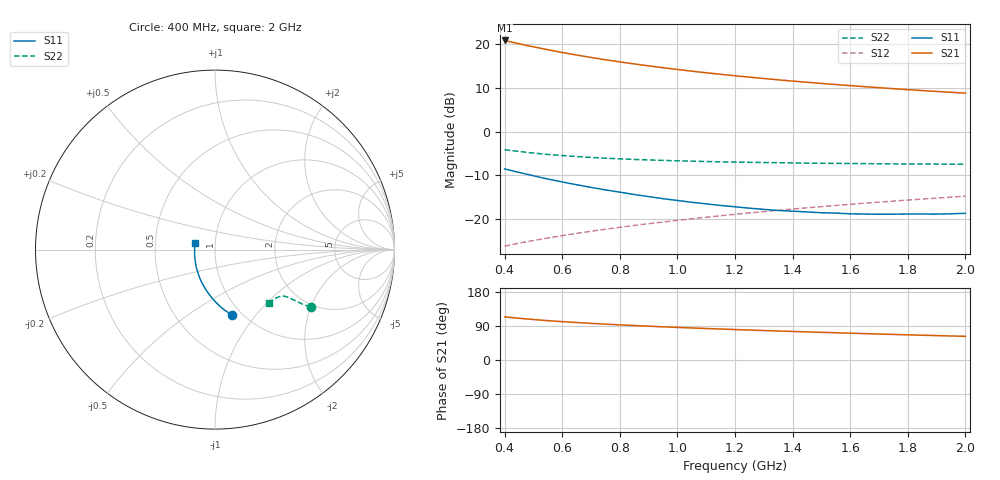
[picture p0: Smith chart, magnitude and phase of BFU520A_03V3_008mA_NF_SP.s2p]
! Filename:  P:\Prog\Test\Noise\ATS_data\Testdata_Net\06 Compressed Noise after Statistics\BFU520A_APG2013_30_A05_03p3V_008mA_NF_CM01_D.sf
! Date/Time: Wed 24/Apr/2013 20:06:16
! BFU520A_APG2013_30_A05_03p3V_1to20mA_NF_CM01_Bias5_R.sf
! Noise Parameter Data File
! BFU520A_APG2013_30_A05_03p3V_1to20mA_NF_CM01
! Date/time: Thu Apr 11 00:04:13 2013
! VAR V_out= 3.300000
! VAR I_out= 7.995000
! VAR V_in= 0.843200
! VAR I_in= 0.090005
! Device data file deembeded for feedlines and parallel
! Original file: \06 Compressed Noise after Statistics\BFU520A_APG2013_30_A05_03p3V_008mA_NF_CM01_R.sf
! Feed-files: PR017V01_150413_Feed1.s2p, PR017V01_150413_Feed2.s2p
! Parallel-file: PR017V01_150413_Par.s2p
# MHz S MA R 50
!  Freq-MHz  S11-mag  S11-arg  S21-mag  S21-arg  S12-mag  S12-arg  S22-mag  S22-arg
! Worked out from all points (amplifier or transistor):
!   37 points, 400 MHz to 2 GHz, reference 50 ohm
!   highest |S21| = 20.9 dB at 400 MHz (marker M1)
!   |S21| within 3 dB of that: start of sweep to 621.3 MHz
!   unconditionally stable (mu >= 1): 1.331 GHz to end of sweep
!   at 500 MHz: K = 0.78, MSG = 22.2 dB, |S12| = -24.9 dB
!   at 1.1 GHz: K = 0.98, MSG = 16.5 dB, |S12| = -19.6 dB
!   at 2 GHz: K = 1.01, MAG = 11.2 dB, |S12| = -14.8 dB
!   lowest NFmin = 0.77 dB at 420 MHz
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400  0.3744 -75.7  11.06 113.9  0.04886 66.5  0.621 -31.0
420  0.361 -77.8  10.67 112.3  0.05052 66.4  0.6089 -31.3
440  0.3475 -79.9  10.31 110.8  0.05208 66.4  0.598 -31.5
460  0.3356 -81.8  9.965 109.5  0.05367 66.4  0.5879 -31.7
480  0.324 -83.8  9.645 108.2  0.0552 66.5  0.5777 -31.9
500  0.3125 -85.8  9.341 106.9  0.05679 66.5  0.5693 -32.0
550  0.2868 -90.3  8.674 103.8  0.06059 66.8  0.5482 -32.2
600  0.2653 -94.5  8.057 101.2  0.06453 67.0  0.5323 -32.4
650  0.2468 -98.5  7.532 98.9  0.06843 67.3  0.5185 -32.6
700  0.2302 -102.5  7.069 96.7  0.07236 67.6  0.5068 -32.7
750  0.2154 -106.2  6.653 94.6  0.07633 67.9  0.4967 -32.9
800  0.2029 -110.2  6.288 92.7  0.08036 68.1  0.4884 -33.1
850  0.1907 -114.1  5.959 90.9  0.08437 68.3  0.4806 -33.3
950  0.1708 -121.6  5.39 87.5  0.09243 68.7  0.4684 -33.8
1050  0.1553 -128.9  4.923 84.5  0.1006 68.9  0.4587 -34.4
1150  0.1429 -136.9  4.533 81.7  0.1089 69.0  0.4511 -35.1
1200  0.1379 -140.5  4.362 80.4  0.1131 69.0  0.4482 -35.5
1350  0.1251 -152.2  3.918 76.5  0.1258 69.0  0.441 -36.8
1500  0.118 -163.9  3.562 73.0  0.1386 68.7  0.4343 -38.3
1650  0.114 -174.7  3.272 69.6  0.1517 68.3  0.4304 -40.1
1750  0.1135 178.0  3.102 67.4  0.1603 68.0  0.4276 -41.3
2000  0.1163 162.4  2.759 62.4  0.1824 67.0  0.4229 -44.7
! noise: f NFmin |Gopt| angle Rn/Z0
400  0.8033  0.04943  34.64  0.111
460  0.8049  0.03047  42.78  0.0993
600  0.8846  0.04723  21.37  0.1195
800  0.8413  0.0284  141.3  0.0954
1000  0.8857  0.0323  137.8  0.0937
1200  0.904  0.04245  158.3  0.0982
1400  0.9252  0.05861  -177  0.1045
1600  0.9388  0.08401  -160.4  0.0916
1800  0.9522  0.1355  -161.8  0.0785
2000  0.9359  0.1235  -135.8  0.101
